FUNCTION_BLOCK Example34_RotaryMotion //1x1 flyways 1 xbots - SingleAxisMotion,RotaryMotion,RotaryMotionSpin
VAR_INPUT
	Execute : BOOL;
END_VAR
VAR_OUTPUT
	Done : BOOL;
END_VAR
VAR_IN_OUT
	PM_Controller : PMControllerType;	// the planar motor controller to use
END_VAR
VAR
	PMC_SingleAxisMotion0 : PMC_SingleAxisMotion;
	PMC_SingleAxisMotion1 : PMC_SingleAxisMotion;
	PMC_SingleAxisMotion2 : PMC_SingleAxisMotion;
	PMC_RotaryMotion0 : PMC_RotaryMotion;
	PMC_RotaryMotionSpin0 : PMC_RotaryMotionSpin; 
	PI : REAL := 3.14159265;
END_VAR

//1x1 flyways 1 xbots - SingleAxisMotion,RotaryMotion,RotaryMotionSpin

//move xbot 1 to x = 120 mm
PMC_SingleAxisMotion0(Execute := Execute,cmdLB := 0,XbotID := 1,Mode := 0,Priority := 0,AxisID := 1,Pos := 0.12,EndVel := 0,MaxVel := 1,MaxAcc := 10,PM_Controller := PM_Controller);

//move xbot 1 to y = 180 mm
PMC_SingleAxisMotion1(Execute := PMC_SingleAxisMotion0.Done,cmdLB := 0,XbotID := 1,Mode := 0,Priority := 0,AxisID := 2,Pos := 0.18,EndVel := 0,MaxVel := 1,MaxAcc := 10,PM_Controller := PM_Controller);

//move xbot 1 to down 60 mm in the y axis
PMC_SingleAxisMotion2(Execute := PMC_SingleAxisMotion1.Done,cmdLB := 0,XbotID := 1,Mode := 1,Priority := 0,AxisID := 2,Pos := -0.06,EndVel := 0,MaxVel := 1,MaxAcc := 10,PM_Controller := PM_Controller);

//rotate xbot 1 five times in the positive (counter clockwise) direction
PMC_RotaryMotion0(Execute := PMC_SingleAxisMotion2.Done,cmdLB := 0,XbotID := 1,BoundaryMode := 0,MotionMode := 1,WrapMode := 0,Angle := 10*PI,MaxVel := PI,MaxAcc := 10,PM_Controller := PM_Controller);

//rotate xbot 1 for 10 seconds in the negative (clockwise) direction
PMC_RotaryMotionSpin0(Execute := PMC_RotaryMotion0.Done,cmdLB := 0,XbotID := 1,BoundaryMode := 0,Angle := 0,MaxVel := -PI,MaxAcc := 10,Duration := 10,PM_Controller := PM_Controller);
Done := PMC_RotaryMotionSpin0.Done;

END_FUNCTION_BLOCK
